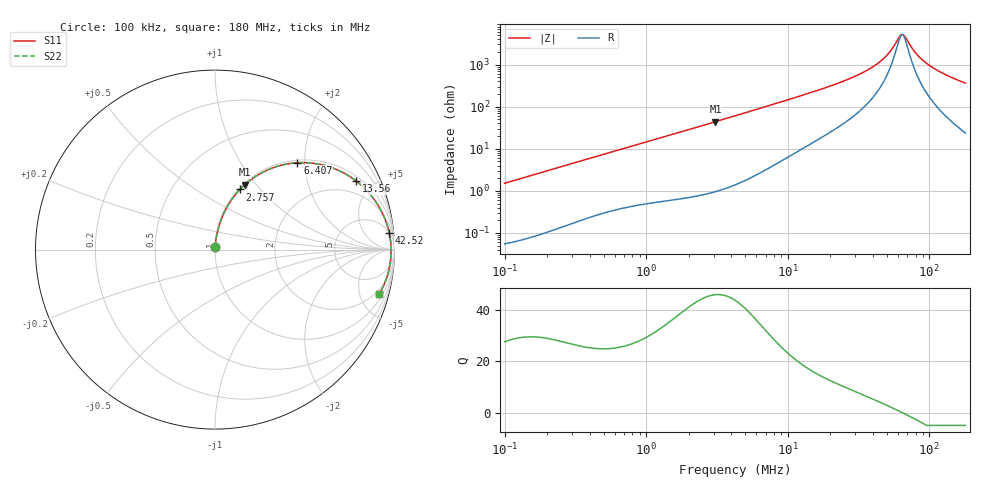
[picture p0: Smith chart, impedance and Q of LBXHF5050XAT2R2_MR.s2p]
! LBXHF5050XAT2R2_MR  S-PARAMETER MODEL  ( General Type )
! Model Generated by TAIYO YUDEN Corporation (http://www.ty-top.com)
! Version 1.0
! TAIYO YUDEN Control No. 201118NI43SB-FBB
! Copyright(c) 2020 TAIYO YUDEN CO.,LTD. All Rights Reserved.
! Product Description (link to TY-COMPAS)
! https://ds.yuden.co.jp/TYCOMPAS/or/detail?pn=LBXHF5050XAT2R2NMR&u=M
! Products Name : Inductors
! Characteristics :
!  Inductance : 2.2 uH , SRF(min) : 45 MHz , DC Resistance(max) : 0.029 Ohm
!  Rated Current : Saturation :5100 mA , Temp Rise : 2500 mA
!  Case Size : 5.0 x 5.0 / 0.197 x 0.197 [mm/inch] , Thickness : 3.1 / 0.122 [mm/inch]
!  (Conditions: Temperature = 25 degC , DC Bias Current/Voltage = 0A / 0V)
! External Node Assignments :
!  1  o---GGG---o  2
! GND o---------o GND
! Frequency Range : 0.1MHz  -  180.004543MHz  [ 402 STEP ]
# MHz S RI R 50
! Freq[MHz].  S11 Real  S11 Imag  S21 Real  S21 Imag  S12 Real  S12 Imag  S22 Real  S22 Imag
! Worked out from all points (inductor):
!   401 points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, 100 kHz to 180 MHz, reference 50 ohm
!   read as one part in series: L = 2.41 uH near 103.8 kHz
!   highest Q = 45.9 at 3.085 MHz (marker M1), where L = 2.27 uH
!   self-resonance near 64.22 MHz
!   S11 on the Smith chart (normalised r, x): 100 kHz: 1.00, +0.03; 2.757 MHz: 1.02, +0.78; 6.407 MHz: 1.05, +1.84; 13.56 MHz: 1.23, +4.00; 42.52 MHz: 5, +20; 180 MHz: 1.47, -7.24
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0.1  0.000778 0.0151  0.9992 -0.0151  0.9992 -0.0151  0.000778 0.0151
0.350962  0.00471 0.0518  0.9953 -0.0518  0.9953 -0.0518  0.00471 0.0518
1.231743  0.0351 0.1693  0.9649 -0.1693  0.9649 -0.1693  0.0351 0.1693
2.757166  0.1389 0.335  0.8611 -0.335  0.8611 -0.335  0.1389 0.335
3.085263  0.1671 0.3623  0.8329 -0.3623  0.8329 -0.3623  0.1671 0.3623
4.322947  0.2802 0.4377  0.7198 -0.4377  0.7198 -0.4377  0.2802 0.4377
6.407407  0.4593 0.484  0.5407 -0.484  0.5407 -0.484  0.4593 0.484
8.977803  0.6233 0.4654  0.3767 -0.4654  0.3767 -0.4654  0.6233 0.4654
13.55847  0.7873 0.3817  0.2127 -0.3817  0.2127 -0.3817  0.7873 0.3817
14.89024  0.8162 0.3576  0.1838 -0.3576  0.1838 -0.3576  0.8162 0.3576
28.15793  0.9391 0.1892  0.0609 -0.1892  0.0609 -0.1892  0.9391 0.1892
35.25813  0.9598 0.1345  0.0402 -0.1345  0.0402 -0.1345  0.9598 0.1345
42.52471  0.9711 0.0912  0.0289 -0.0912  0.0289 -0.0912  0.9711 0.0912
47.58506  0.9756 0.0661  0.0244 -0.0661  0.0244 -0.0661  0.9756 0.0661
52.25907  0.9784 0.0455  0.0216 -0.0455  0.0216 -0.0455  0.9784 0.0455
61.85938  0.9809 0.00882  0.0191 -0.00882  0.0191 -0.00882  0.9809 0.00882
65.43652  0.9811 -0.00336  0.0189 0.00336  0.0189 0.00336  0.9811 -0.00336
67.93547  0.9811 -0.0115  0.0189 0.0115  0.0189 0.0115  0.9811 -0.0115
80.41563  0.9792 -0.0484  0.0208 0.0484  0.0208 0.0484  0.9792 -0.0484
95.18848  0.9742 -0.0864  0.0258 0.0864  0.0258 0.0864  0.9742 -0.0864
126.0833  0.9575 -0.1535  0.0425 0.1535  0.0425 0.1535  0.9575 -0.1535
180.0045  0.9155 -0.2474  0.0845 0.2474  0.0845 0.2474  0.9155 -0.2474
